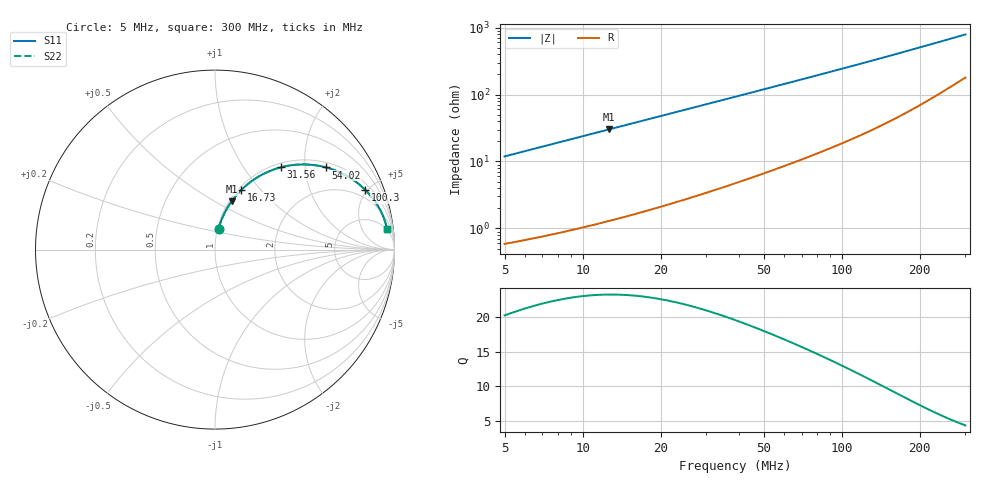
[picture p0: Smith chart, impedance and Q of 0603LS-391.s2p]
# MHz S MA R 50
!Freq  MagS11  AngS11  MagS21  AngS21  MagS12  AngS12  MagS22  AngS22
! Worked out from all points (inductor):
!   801 points, 5 MHz to 300 MHz, reference 50 ohm
!   read as one part in series: L = 379 nH near 5.103 MHz
!   highest Q = 23.3 at 12.63 MHz (marker M1), where L = 379 nH
!   S11 on the Smith chart (normalised r, x): 5 MHz: 1.01, +0.24; 16.73 MHz: 1.03, +0.80; 31.56 MHz: 1.07, +1.50; 54.02 MHz: 1.15, +2.58; 100.3 MHz: 1.37, +4.85; 300 MHz: 5, +15
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5  0.1176 80.4  0.9873 -6.7  0.9873 -6.7  0.1176 80.4
6.591666  0.154 78.5  0.981 -8.8  0.981 -8.8  0.154 78.5
8.298818  0.1923 76.4  0.9729 -11.1  0.9729 -11.1  0.1923 76.4
10.3417  0.2368 73.8  0.9614 -13.7  0.9614 -13.7  0.2368 73.8
12.62632  0.2846 71.0  0.9465 -16.5  0.9465 -16.5  0.2846 71.0
16.7311  0.3647 66.1  0.9154 -21.4  0.9154 -21.4  0.3647 66.1
19.80949  0.4196 62.7  0.8894 -24.8  0.8894 -24.8  0.4196 62.7
23.33455  0.4768 59.0  0.8577 -28.4  0.8577 -28.4  0.4768 59.0
31.56008  0.5878 51.3  0.7812 -36.0  0.7812 -36.0  0.5878 51.3
42.68514  0.6957 43.0  0.6827 -44.0  0.6827 -44.0  0.6957 43.0
54.01575  0.7698 36.5  0.5958 -50.2  0.5958 -50.2  0.7698 36.5
54.29291  0.7713 36.4  0.5939 -50.4  0.5939 -50.4  0.7713 36.4
63.95421  0.8151 32.1  0.5317 -54.4  0.5317 -54.4  0.8151 32.1
74.56754  0.8499 28.2  0.4742 -58.0  0.4742 -58.0  0.8499 28.2
86.49835  0.8779 24.8  0.4208 -61.1  0.4208 -61.1  0.8779 24.8
100.3381  0.9007 21.7  0.3706 -63.9  0.3706 -63.9  0.9007 21.7
103.467  0.9049 21.1  0.3606 -64.4  0.3606 -64.4  0.9049 21.1
125.6794  0.9268 17.5  0.3016 -67.4  0.3016 -67.4  0.9268 17.5
152.6604  0.9425 14.4  0.2497 -69.6  0.2497 -69.6  0.9425 14.4
202.2899  0.9568 10.7  0.187 -71.4  0.187 -71.4  0.9568 10.7
252.0866  0.9627 8.4  0.1477 -71.2  0.1477 -71.2  0.9627 8.4
300  0.9651 6.8  0.1223 -70.0  0.1223 -70.0  0.9651 6.8
